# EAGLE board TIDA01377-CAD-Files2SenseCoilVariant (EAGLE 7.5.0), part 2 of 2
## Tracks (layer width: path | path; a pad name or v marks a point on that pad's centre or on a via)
ADJ
  Top 0.254: R10.2 107.83,35.93 R9.1 | 107.9,35.92 R9.1 | U1.4 107.82,35.17 107.82,35.92 R9.1
AUXVCC1  (via drill 0.2, 0.4)
  Top 0.254: MSP430F67791A.124 120.01,99.28 v121.26,98.03 | v128.51,96.62 C26.1 | C27.1 130.66,94.22 v131.51,93.38
  Top 0.406: C26.1 128.51,93.88 128.86,94.22 C27.1
  Top 0.813: 139.8,90.03 SV1.6
  Bottom 0.254: v128.51,96.62 122.66,96.62 v121.26,98.03
  Bottom 0.61: v131.51,93.38 131.47,93.34 137.36,93.34 SV1.6
AUXVCC2  (via drill 0.2, 0.6)
  Top 0.254: v120.26,98.12 119.51,98.88 MSP430F67791A.123 119.51,108.75 118.59,109.67 114.91,109.67 v114.53,110.05 | C24.1 v125.51,95.62 | v90.02,126.84 88.86,126.84 C58.1 87.27,126.8 R4.2
  Top 0.406: C24.1 125.51,94.38 125.66,94.22 C25.1
  Bottom 0.254: v125.51,95.62 122.76,95.62 v120.26,98.12 | v90.02,126.84 90.04,126.86 107.08,126.86 108.61,125.34 108.61,121.99 109.42,121.17 109.42,118.46 114.53,113.35 v114.53,110.05
  Bottom 0.61: v125.51,95.62 137.61,95.62 SV1.4
AUXVCC3  (via drill 0.3, 0.4)
  Top 0.254: C43.1 128.13,106 | MSP430F67791A.3 124.76,103.38 127.41,106.03 C43.1 | C43.1 128.01,105.88 128.16,106.03 C44.1 130.16,106.03 v131.51,107.38 | v142.76,102.12 142.76,98.62 145.31,96.07 SV1.2 148.51,90.47 D44.C
  Bottom 0.254: v131.51,107.38 138.81,107.38 142.71,103.47 142.71,102.17 v142.76,102.12 142.81,102.07
AVCC
  Top 0.254: 117.76,94.62 117.86,94.53 C29.1 | 118.01,95.88 117.96,95.83 C31.1 | MSP430F67791A.121 118.51,99.2 118.01,98.7 118.01,95.83 C31.1 | C31.1 117.81,95.83 117.76,95.88 117.91,96.03
  Top 0.406: C29.1 118.01,94.62 117.91,94.72
  Top 0.61: 117.91,94.72 C31.1 | 117.86,94.53 117.86,89.22 119.2,87.89 R36.2
BTN1  (via drill 0.6)
  Top 0.254: MSP430F67791A.7 124.86,105.38 125.19,105.71 125.19,111.34 127.23,113.38 v128.83,113.38 | v136.51,115.88 136.51,125.22 139.56,128.28 R53.2
  Top 0.406: R53.2 139.56,137.29 DBTN1.2
  Bottom 0.254: v128.83,113.38 134.01,113.38 v136.51,115.88 | 140.01,137.74 DBTN1.2
BTN2
  Top 0.254: MSP430F67791A.6 125.1,104.88 125.96,105.73 125.96,110.63 127.33,112 130.22,112 133.6,115.38 133.6,115.41 135.28,117.08 135.28,130.98 133.83,132.43 131.94,132.43 R50.2 131.89,136.36 DBTN2.2
COILS  (via drill 0.36 pad 0.58, 1.02 pad 1.52)
  Top 0.254: R12.2 v118.44,29.86 118.49,29.91 139.16,29.91 151.41,42.16 151.41,139.21 144.57,146.04 144.57,153.64 144.5,153.64 141.24,153.66 138.11,154.52 135.31,156.16 133.04,158.47 131.44,161.28 130.62,164.4 130.65,167.62 131.5,170.72 133.12,173.49 135.4,175.74 138.18,177.32 141.27,178.13 144.46,178.11 147.53,177.26 150.27,175.66 152.5,173.4 154.06,170.65 154.86,167.59 154.84,164.44 154,161.4 152.41,158.69 150.18,156.48 147.46,154.94 144.43,154.15 141.31,154.17 138.31,155 135.62,156.57 133.44,158.78 131.91,161.47 131.13,164.47 131.15,167.55 131.97,170.52 133.53,173.18 135.71,175.34 138.38,176.85 141.34,177.62 144.39,177.6 147.33,176.79 149.96,175.25 152.09,173.09 153.59,170.45 154.35,167.52 154.33,164.5 153.53,161.59 152.01,159 149.87,156.89 147.26,155.41 144.36,154.66 141.38,154.68 138.5,155.47 135.94,156.97 133.85,159.09 132.39,161.67 131.64,164.53 131.66,167.49 132.44,170.33 133.93,172.87 136.03,174.93 138.58,176.38 141.41,177.11 144.33,177.09 147.14,176.32 149.65,174.84 151.69,172.78 153.12,170.25 153.84,167.46 153.82,164.57 153.06,161.79 151.6,159.31 149.56,157.3 147.06,155.88 144.3,155.16 141.44,155.18 138.7,155.94 136.25,157.38 134.26,159.4 132.86,161.86 132.15,164.6 132.17,167.42 132.92,170.13 134.34,172.55 136.34,174.52 138.77,175.9 141.47,176.6 144.26,176.58 146.94,175.84 149.33,174.44 151.28,172.46 152.64,170.06 153.34,167.39 153.31,164.63 152.58,161.99 151.19,159.62 149.24,157.7 146.87,156.36 144.23,155.67 141.51,155.69 138.89,156.41 136.56,157.79 134.66,159.71 133.33,162.06 132.66,164.67 132.68,167.35 133.39,169.94 134.75,172.24 136.65,174.12 138.97,175.43 141.54,176.1 144.19,176.07 146.75,175.37 149.02,174.03 150.87,172.15 152.17,169.86 152.83,167.32 152.81,164.7 152.11,162.18 150.79,159.94 148.93,158.11 146.67,156.83 144.16,156.18 141.58,156.2 139.09,156.89 136.87,158.19 135.07,160.03 133.81,162.26 133.16,164.73 133.19,167.29 133.87,169.74 135.15,171.93 136.96,173.71 139.16,174.96 141.61,175.59 144.13,175.57 146.55,174.9 148.71,173.62 150.47,171.84 151.7,169.67 152.32,167.25 152.3,166.01 v151.74,166.01
  Top 0.254: 115.17,32.38 R13.2 115.15,32.4 v118.44,32.4 130.38,32.4 131.24,33.27 131.24,36.17 131.95,36.88 134.6,36.9 137.73,37.76 140.53,39.4 142.8,41.7 144.4,44.51 145.22,47.64 145.19,50.86 144.34,53.96 142.72,56.73 140.44,58.98 137.66,60.56 134.57,61.37 131.38,61.34 128.31,60.5 125.57,58.89 123.34,56.63 121.78,53.88 120.98,50.83 121,47.67 121.84,44.64 123.43,41.92 125.66,39.72 128.38,38.17 131.41,37.38 134.53,37.4 137.53,38.23 140.22,39.8 142.4,42.01 143.93,44.71 144.71,47.7 144.69,50.79 143.87,53.76 142.31,56.41 140.13,58.57 137.46,60.09 134.5,60.86 131.44,60.84 128.51,60.03 125.88,58.49 123.75,56.32 122.25,53.69 121.49,50.76 121.51,47.74 122.31,44.83 123.83,42.23 125.97,40.13 128.58,38.64 131.48,37.89 134.46,37.91 137.34,38.7 139.9,40.21 141.99,42.33 143.45,44.9 144.2,47.77 144.18,50.72 143.39,53.56 141.91,56.1 139.81,58.16 137.26,59.61 134.43,60.35 131.51,60.33 128.7,59.55 126.19,58.08 124.15,56.01 122.72,53.49 122,50.69 122.02,47.8 122.78,45.03 124.24,42.55 126.28,40.53 128.78,39.12 131.54,38.4 134.4,38.42 137.14,39.18 139.59,40.62 141.58,42.64 142.98,45.1 143.69,47.84 143.67,50.66 142.92,53.37 141.5,55.79 139.5,57.76 137.07,59.14 134.37,59.84 131.58,59.82 128.9,59.08 126.5,57.67 124.56,55.7 123.2,53.3 122.5,50.62 122.52,47.87 123.26,45.22 124.65,42.86 126.6,40.94 128.97,39.59 131.61,38.91 134.33,38.93 136.95,39.65 139.28,41.02 141.18,42.95 142.51,45.3 143.18,47.9 143.16,50.59 142.45,53.17 141.09,55.48 139.19,57.35 136.87,58.66 134.3,59.33 131.65,59.31 129.09,58.61 126.82,57.27 124.97,55.39 123.67,53.1 123.01,50.56 123.03,47.94 123.73,45.42 125.05,43.17 126.91,41.34 129.17,40.06 131.68,39.41 134.26,39.44 136.75,40.12 138.97,41.43 140.77,43.26 142.03,45.49 142.68,47.97 142.65,50.52 141.97,52.98 140.69,55.17 138.88,56.95 136.68,58.19 134.23,58.83 131.71,58.8 129.29,58.13 127.13,56.86 125.37,55.08 124.14,52.9 123.52,50.49 123.54,48 124.2,45.61 125.46,43.48 127.22,41.75 129.36,40.54 131.74,39.92 134.2,39.94 136.55,40.6 138.66,41.84 140.36,43.57 141.56,45.69 142.17,48.04 142.15,50.45 141.5,52.78 140.28,54.85 138.57,56.54 136.48,57.72 134.16,58.32 131.78,58.3 129.49,57.66 127.44,56.45 125.78,54.76 124.62,52.71 124.03,50.42 124.05,48.07 124.68,45.81 125.87,43.8 127.53,42.16 129.56,41.01 131.81,40.43 134.13,40.45 136.36,41.07 138.34,42.24 139.96,43.89 141.09,45.89 141.66,48.1 141.64,50.39 141.03,52.58 139.87,54.54 138.25,56.13 136.28,57.24 134.1,57.81 131.85,57.79 129.68,57.19 127.75,56.05 126.19,54.45 125.09,52.51 124.54,50.36 124.56,48.14 125.15,46.01 126.27,44.11 127.84,42.56 129.76,41.48 131.88,40.94 134.06,40.96 136.16,41.54 138.03,42.65 139.55,44.2 140.61,46.08 141.15,48.17 141.13,50.32 140.55,52.39 139.47,54.23 137.94,55.73 136.09,56.77 134.03,57.3 131.91,57.28 129.88,56.71 128.06,55.64 126.59,54.14 125.56,52.31 125.04,50.29 125.06,48.21 125.62,46.2 126.68,44.42 128.16,42.97 129.95,41.96 131.94,41.45 133.99,41.47 135.96,42.02 137.72,43.06 139.14,44.51 140.14,46.28 140.64,48.24 140.62,50.25 140.08,52.19 139.06,53.92 137.63,55.32 135.89,56.3 133.96,56.79 131.98,56.77 130.07,56.24 128.38,55.23 127,53.83 126.04,52.12 125.55,50.22 125.57,49.25 v126.13,49.25 v126.13,49.24
  Top 0.254: R11.2 118.36,27.25 v118.44,27.32 | v124.1,13.15 v124.1,13.14 123.54,13.14 123.52,11.9 124.14,9.49 125.37,7.31 127.13,5.53 129.29,4.26 131.71,3.59 134.23,3.57 136.68,4.2 138.88,5.45 140.69,7.22 141.97,9.41 142.65,11.87 142.68,14.42 142.03,16.9 140.77,19.13 138.97,20.96 136.75,22.27 134.26,22.95 131.68,22.98 129.17,22.32 126.91,21.05 125.05,19.22 123.73,16.97 123.03,14.45 123.01,11.83 123.67,9.29 124.97,7 126.82,5.12 129.09,3.79 131.65,3.08 134.3,3.06 136.87,3.73 139.19,5.04 141.09,6.91 142.45,9.22 143.16,11.8 143.18,14.49 142.51,17.09 141.18,19.44 139.28,21.37 136.95,22.74 134.33,23.46 131.61,23.48 128.97,22.8 126.6,21.45 124.65,19.53 123.26,17.17 122.52,14.52 122.5,11.77 123.2,9.1 124.56,6.69 126.5,4.72 128.9,3.31 131.58,2.57 134.37,2.55 137.07,3.25 139.5,4.63 141.5,6.6 142.92,9.02 143.67,11.73 143.69,14.55 142.98,17.29 141.58,19.75 139.59,21.77 137.14,23.21 134.4,23.97 131.54,23.99 128.78,23.27 126.28,21.86 124.24,19.84 122.78,17.36 122.02,14.59 122,11.7 122.72,8.9 124.15,6.38 126.19,4.31 128.7,2.84 131.51,2.06 134.43,2.04 137.26,2.78 139.81,4.23 141.91,6.29 143.39,8.83 144.18,11.67 144.2,14.62 143.45,17.49 141.99,20.06 139.9,22.18 137.34,23.69 134.46,24.48 131.48,24.5 128.58,23.75 125.97,22.27 123.83,20.16 122.31,17.56 121.51,14.65 121.49,11.63 122.25,8.7 123.75,6.07 125.88,3.9 128.51,2.36 131.44,1.55 134.5,1.53 137.46,2.3 140.13,3.82 142.31,5.98 143.87,8.63 144.69,11.6 144.71,14.69 143.93,17.68 142.4,20.38 140.22,22.59 137.53,24.16 134.53,24.99 131.41,25.01 128.38,24.22 125.66,22.67 123.43,20.47 121.84,17.76 121,14.72 120.98,11.57 121.78,8.51 123.34,5.76 125.57,3.5 128.31,1.89 131.38,1.05 134.57,1.03 137.66,1.83 140.44,3.41 142.72,5.66 144.34,8.43 145.19,11.54 145.22,14.76 144.4,17.88 142.8,20.69 140.53,22.99 137.73,24.63 134.6,25.5 131.34,25.52 131.27,25.52 131.27,26.53 131.72,26.99 v132.48,26.99
  Bottom 0.254: v120.47,27.32 120.47,13.14 120.49,11.5 121.36,8.34 123.02,5.51 125.35,3.21 128.19,1.59 131.34,0.77 134.6,0.79 137.73,1.65 140.53,3.29 142.8,5.6 144.4,8.41 145.22,11.53 145.19,14.75 144.34,17.85 142.72,20.62 140.44,22.87 137.66,24.46 134.57,25.26 131.38,25.24 128.31,24.4 125.57,22.79 123.34,20.53 121.78,17.78 120.98,14.72 121,11.57 121.84,8.53 123.43,5.82 125.66,3.62 128.38,2.07 131.41,1.28 134.53,1.3 137.53,2.13 140.22,3.7 142.4,5.91 143.93,8.61 144.71,11.6 144.69,14.69 143.87,17.66 142.31,20.31 140.13,22.47 137.46,23.98 134.5,24.75 131.44,24.73 128.51,23.92 125.88,22.38 123.75,20.22 122.25,17.58 121.49,14.66 121.51,11.63 122.31,8.73 123.83,6.13 125.97,4.02 128.58,2.54 131.48,1.79 134.46,1.81 137.34,2.6 139.9,4.11 141.99,6.22 143.45,8.8 144.2,11.66 144.18,14.62 143.39,17.46 141.91,20 139.81,22.06 137.26,23.51 134.43,24.25 131.51,24.22 128.7,23.45 126.19,21.98 124.15,19.91 122.72,17.39 122,14.59 122.02,11.7 122.78,8.92 124.24,6.44 126.28,4.43 128.78,3.02 131.54,2.3 134.4,2.32 137.14,3.07 139.59,4.51 141.58,6.54 142.98,9 143.69,11.73 143.67,14.55 142.92,17.27 141.5,19.69 139.5,21.66 137.07,23.04 134.37,23.74 131.58,23.72 128.9,22.98 126.5,21.57 124.56,19.6 123.2,17.19 122.5,14.52 122.52,11.77 123.26,9.12 124.65,6.76 126.6,4.84 128.97,3.49 131.61,2.8 134.33,2.82 136.95,3.55 139.28,4.92 141.18,6.85 142.51,9.19 143.18,11.8 143.16,14.49 142.45,17.07 141.09,19.38 139.19,21.25 136.87,22.56 134.3,23.23 131.65,23.21 129.09,22.5 126.82,21.16 124.97,19.29 123.67,17 123.01,14.46 123.03,11.84 123.73,9.32 125.05,7.07 126.91,5.24 129.17,3.96 131.68,3.31 134.26,3.33 136.75,4.02 138.97,5.33 140.77,7.16 142.03,9.39 142.68,11.87 142.65,14.42 141.97,16.87 140.69,19.06 138.88,20.84 136.68,22.09 134.23,22.72 131.71,22.7 129.29,22.03 127.13,20.76 125.37,18.97 124.14,16.8 123.52,14.39 123.54,13.14 v124.1,13.14 v124.1,13.15
  Bottom 0.254: v120.47,27.32 v118.44,27.32 | v120.47,27.32 | v151.74,166.01 152.3,166.01 152.32,164.77 151.7,162.35 150.47,160.18 148.71,158.4 146.55,157.12 144.13,156.45 141.61,156.43 139.16,157.07 136.96,158.31 135.15,160.09 133.87,162.28 133.19,164.74 133.16,167.29 133.81,169.76 135.07,172 136.87,173.83 139.09,175.13 141.58,175.82 144.16,175.84 146.67,175.19 148.93,173.91 150.79,172.09 152.11,169.84 152.81,167.32 152.83,164.7 152.17,162.16 150.87,159.87 149.02,157.99 146.75,156.65 144.19,155.95 141.54,155.93 138.97,156.59 136.65,157.91 134.75,159.78 133.39,162.09 132.68,164.67 132.66,167.35 133.33,169.96 134.66,172.31 136.56,174.23 138.89,175.61 141.51,176.33 144.23,176.35 146.87,175.67 149.24,174.32 151.19,172.4 152.58,170.03 153.31,167.39 153.34,164.63 152.64,161.96 151.28,159.56 149.33,157.58 146.94,156.18 144.26,155.44 141.47,155.42 138.77,156.12 136.34,157.5 134.34,159.47 132.92,161.89 132.17,164.6 132.15,167.42 132.86,170.16 134.26,172.62 136.25,174.64 138.7,176.08 141.44,176.84 144.3,176.86 147.06,176.14 149.56,174.72 151.6,172.71 153.06,170.23 153.82,167.45 153.84,164.57 153.12,161.77 151.69,159.25 149.65,157.18 147.14,155.71 144.33,154.93 141.41,154.91 138.58,155.65 136.03,157.09 133.93,159.16 132.44,161.69 131.66,164.53 131.64,167.49 132.39,170.35 133.85,172.93 135.94,175.05 138.5,176.55 141.38,177.34 144.36,177.37 147.26,176.61 149.87,175.13 152.01,173.02 153.53,170.43 154.33,167.52 154.35,164.5 153.59,161.57 152.09,158.93 149.96,156.77 147.33,155.23 144.39,154.42 141.34,154.4 138.38,155.17 135.71,156.69 133.53,158.84 131.97,161.5 131.15,164.47 131.13,167.56 131.91,170.55 133.44,173.24 135.62,175.45 138.31,177.03 141.31,177.85 144.43,177.88 147.46,177.09 150.18,175.54 152.41,173.33 154,170.62 154.84,167.59 154.86,164.43 154.06,161.37 152.5,158.62 150.27,156.37 147.53,154.76 144.46,153.91 141.27,153.89 138.18,154.7 135.4,156.28 133.12,158.53 131.5,161.3 130.65,164.4 130.62,167.62 131.44,170.75 133.04,173.56 135.31,175.86 138.11,177.5 141.24,178.36 144.5,178.38 147.65,177.56 150.49,175.94 152.82,173.65 154.48,170.82 155.35,167.65 155.37,166.01 155.37,151.83 155.37,40.1 142.26,26.99 v132.48,26.99
  Bottom 0.254: v126.13,49.24 v126.13,49.25 125.57,49.25 125.55,48.27 126.04,46.38 127,44.67 128.38,43.26 130.07,42.25 131.98,41.72 133.96,41.7 135.89,42.2 137.63,43.17 139.06,44.58 140.08,46.3 140.62,48.24 140.64,50.26 140.14,52.22 139.14,53.98 137.72,55.44 135.96,56.48 133.99,57.03 131.94,57.05 129.95,56.53 128.16,55.52 126.68,54.08 125.62,52.29 125.06,50.29 125.04,48.2 125.56,46.18 126.59,44.35 128.06,42.85 129.88,41.78 131.91,41.21 134.03,41.19 136.09,41.72 137.94,42.77 139.47,44.26 140.55,46.11 141.13,48.17 141.15,50.32 140.61,52.41 139.55,54.3 138.03,55.84 136.16,56.95 134.06,57.53 131.88,57.55 129.76,57.01 127.84,55.93 126.27,54.39 125.15,52.49 124.56,50.35 124.54,48.14 125.09,45.98 126.19,44.04 127.75,42.45 129.68,41.31 131.85,40.71 134.1,40.69 136.28,41.25 138.25,42.36 139.87,43.95 141.03,45.91 141.64,48.11 141.66,50.39 141.09,52.61 139.96,54.61 138.34,56.25 136.36,57.42 134.13,58.04 131.81,58.06 129.56,57.48 127.53,56.34 125.87,54.7 124.68,52.68 124.05,50.42 124.03,48.07 124.62,45.79 125.78,43.73 127.44,42.04 129.49,40.83 131.78,40.2 134.16,40.18 136.48,40.77 138.57,41.95 140.28,43.64 141.5,45.71 142.15,48.04 142.17,50.46 141.56,52.8 140.36,54.92 138.66,56.66 136.55,57.9 134.2,58.55 131.74,58.57 129.36,57.95 127.22,56.74 125.46,55.01 124.2,52.88 123.54,50.49 123.52,48 124.14,45.59 125.37,43.42 127.13,41.63 129.29,40.36 131.71,39.69 134.23,39.67 136.68,40.3 138.88,41.55 140.69,43.33 141.97,45.52 142.65,47.97 142.68,50.52 142.03,53 140.77,55.23 138.97,57.06 136.75,58.37 134.26,59.06 131.68,59.08 129.17,58.43 126.91,57.15 125.05,55.32 123.73,53.08 123.03,50.55 123.01,47.94 123.67,45.39 124.97,43.11 126.82,41.23 129.09,39.89 131.65,39.18 134.3,39.16 136.87,39.83 139.19,41.14 141.09,43.02 142.45,45.32 143.16,47.91 143.18,50.59 142.51,53.2 141.18,55.54 139.28,57.47 136.95,58.84 134.33,59.57 131.61,59.59 128.97,58.9 126.6,57.55 124.65,55.63 123.26,53.27 122.52,50.62 122.5,47.87 123.2,45.2 124.56,42.79 126.5,40.82 128.9,39.41 131.58,38.67 134.37,38.65 137.07,39.36 139.5,40.74 141.5,42.7 142.92,45.12 143.67,47.84 143.69,50.66 142.98,53.39 141.58,55.86 139.59,57.88 137.14,59.32 134.4,60.07 131.54,60.09 128.78,59.38 126.28,57.96 124.24,55.95 122.78,53.47 122.02,50.69 122,47.8 122.72,45 124.15,42.48 126.19,40.41 128.7,38.94 131.51,38.17 134.43,38.14 137.26,38.88 139.81,40.33 141.91,42.39 143.39,44.93 144.18,47.77 144.2,50.73 143.45,53.59 141.99,56.17 139.9,58.28 137.34,59.79 134.46,60.58 131.48,60.6 128.58,59.85 125.97,58.37 123.83,56.26 122.31,53.66 121.51,50.76 121.49,47.73 122.25,44.81 123.75,42.17 125.88,40.01 128.51,38.47 131.44,37.66 134.5,37.64 137.46,38.41 140.13,39.92 142.31,42.08 143.87,44.73 144.69,47.7 144.71,50.79 143.93,53.78 142.4,56.48 140.22,58.69 137.53,60.26 134.53,61.09 131.41,61.11 128.38,60.32 125.66,58.77 123.43,56.57 121.84,53.86 121,50.82 120.98,47.67 121.78,44.61 123.34,41.86 125.57,39.6 128.31,37.99 131.38,37.15 134.57,37.13 137.66,37.94 140.44,39.52 142.72,41.77 144.34,44.54 145.19,47.64 145.22,50.86 144.4,53.98 142.8,56.79 140.53,59.1 137.73,60.74 134.6,61.6 131.34,61.62 128.19,60.8 125.35,59.18 123.02,56.88 121.36,54.05 120.49,50.89 120.47,50.87 120.47,49.25 v120.47,27.32
COM0  (via drill 0.2)
  Top 0.254: MSP430F67791A.22 121.01,112.88 v113.51,120.38 | LCD1.COM0 94.38,171.5 v109.26,156.62
  Bottom 0.254: v113.51,120.38 113.51,152.38 v109.26,156.62
COM1  (via drill 0.2)
  Top 0.254: MSP430F67791A.23 121.51,113.38 v114.51,120.38 | v109.26,158.12 109.26,158.15 96.62,170.78 96.62,171.46 LCD1.COM1
  Bottom 0.254: v114.51,120.38 114.51,152.88 v109.26,158.12
COM2  (via drill 0.2)
  Top 0.254: MSP430F67791A.24 122.01,113.88 v115.51,120.38 | LCD1.COM2 99.2,169.68 v109.26,159.62
  Bottom 0.254: v115.51,120.38 115.51,153.38 v109.26,159.62
COM3  (via drill 0.2)
  Top 0.254: MSP430F67791A.25 122.51,114.38 v116.51,120.38 | v109.26,161.12 109.26,161.19 101.7,168.75 101.7,171.46 LCD1.COM3
  Bottom 0.254: v116.51,120.38 116.51,153.88 v109.26,161.12
DRESET  (via drill 0.36)
  Top 0.254: v49.01,129.88 49.51,129.38 89.51,129.38 91.01,127.88 91.01,111.77 v91.03,111.75 | MSP430F67791A.102 106.51,102.38 v104.63,100.5
  Bottom 0.254: JP5.2 27.99,136.81 42.08,136.81 v49.01,129.88 | v104.63,100.5 96.38,100.5 91.13,105.75 91.13,111.65 v91.03,111.75
DRV4GND
  Top 0.254: MSP430F67791A.95 95.09,105.88 90.63,101.41 90.63,84.78 90.09,84.24 67.21,84.24 66.57,84.88 66.57,85.97 65.7,86.84 U4GND.1
DRV5GND
  Top 0.254: MSP430F67791A.93 94.16,106.88 89.46,102.18 89.46,88.28 87.98,86.81 U5GND.1
DRV6GND
  Top 0.254: MSP430F67791A.88 93.51,109.38 87.35,103.22 87.35,95.98 85.77,94.4 78.36,94.4 75.39,97.38 75.39,100.53 73.33,102.58 68.2,102.58 67.41,101.8 67.41,100.67 U6GND.1
DRV456OUTA  (via drill 0.5, 0.6)
  Top 0.254: MSP430F67791A.89 93.74,108.88 87.93,103.06 87.93,94.66 86.76,93.49 78.36,93.49 v78.1,93.23 78.03,93.31 75.84,93.31 75.79,93.36 75.77,93.36 73.73,95.39 73.73,99.05 73.19,99.6 U6OUT.1 | U5OUT.1 83.44,90.44 v84.4,89.48
  Top 0.305: U4OUT.1 59.67,83.44 v59.97,83.15 | 79.82,90.42 U5OUT.1
  Bottom 0.254: v59.97,83.15 75.16,83.15 | v84.4,89.48 84.4,84.09 83.46,83.15 75.16,83.15 | 75.16,83.15 75.61,83.61 75.61,92.35 76.58,93.31 78.03,93.31 v78.1,93.23
DRV456OUTB
  Top 0.254: MSP430F67791A.94 94.62,106.38 89.99,101.74 89.99,85.13 89.56,84.7 69.59,84.7 69.19,85.11 U$8.3
DRVOUT4  (via drill 0.5, 0.6)
  Top 0.254: U$8.1 | 70.86,83.79 65.56,83.79 65.02,84.32 65.02,85.21 | 70.86,83.79 109.75,83.79 v110.08,84.12 | v114.45,106.29 118.31,106.29 v118.36,106.24 | v121.54,106.24 122.2,106.24 122.33,106.38 MSP430F67791A.9 | 68.03,79.15 R17.1 69.75,79.15 C12.1 69.67,79.23 69.67,80.87 70.15,81.35 70.15,83.08 70.86,83.79
  Top 0.305: U$8.1 68.17,85.36 v68.02,85.21 | v65.48,85.21 65.02,85.21
  Bottom 0.254: v110.08,84.12 110.08,101.92 v114.45,106.29 | v118.36,106.24 v121.54,106.24
  Bottom 0.305: v68.02,85.21 v65.48,85.21
DRVOUT5  (via drill 0.6)
  Top 0.254: 86.15,91.58 v86.21,91.53 86,91.74 72.06,91.74 71.17,90.85 71.17,89.3 71.65,88.81 72.61,88.81 C14.1 72.58,88.64 72.58,86.99 R16.1 71.55,86.94 | MSP430F67791A.10 123.78,106.85 122.12,106.85 v121.51,107.46 | v118.26,107.46 115.57,107.46 115.34,107.69 114.5,107.69 v114.48,107.66
  Top 0.305: U$8.2 68.68,86.66 68.96,86.94 71.55,86.94
  Bottom 0.254: v86.21,91.53 90.32,91.53 97,84.85 108.71,84.85 109.55,85.69 109.55,102.73 v114.48,107.66 | v121.51,107.46 v118.26,107.46
DRVOUT6  (via drill 0.6)
  Top 0.254: v117.96,108.63 113.61,108.63 v113.59,108.6 | U$8.5 69.68,92.96 R15.1 69.63,93.03 71.63,93.03 72.31,92.35 87.96,92.35 v88.19,92.57 | MSP430F67791A.11 123.02,107.38 v121.79,108.6
  Top 0.305: R15.1 67.82,93.02 C15.1
  Bottom 0.254: v117.96,108.63 117.98,108.6 v121.79,108.6 | v113.59,108.6 113.59,108.55 108.61,103.57 108.61,93.56 107.11,92.07 105.26,92.07 104.75,92.57 v88.19,92.57
DRVPOWER1
  Top 0.61: R1.1 28.88,191.68 28.88,190.44 28.37,189.93 DRV_U$7.1 22.85,189.9 U$7.1 18.82,189.9 18.57,190.16 18.57,193.96 C1.1
DRVPOWER4  (via drill 0.5)
  Top 0.254: v60.93,92.45 64.11,92.45 66.25,90.3 R68.2
  Top 0.61: 59.25,89.58 R45.1 | R45.1 59.11,89.8 | v60.93,92.45 60.45,91.96 C52.1 59.5,91.14 59.1,90.75 59.1,89.44 R45.1 | U$4.1 59.24,89.3 R45.1
  Bottom 0.305: 71.34,100.16 R64.1
  Bottom 0.61: 82.14,95.72 85.14,95.72 87.32,97.91 DRV-I1.1 | C54.1 81.03,88.37 U$5.1 80.62,89.94 80.67,89.98 R47.1 80.31,90.56 80.31,93.89 82.14,95.72 | 71.34,100.16 U$6.1 68.74,100.72 C55.1 62.83,100.72 60.96,98.85 60.96,92.47 v60.93,92.45 | R64.1 71.55,100.17 73.05,100.17 74.88,98.33 74.88,96.16 75.32,95.72 82.14,95.72
DRVU7  (via drill 0.6)
  Top 0.254: R1.2 27.04,192.87 28.55,194.38 32.05,194.38 39.14,187.29 39.14,163.09 v57.4,144.82 | MSP430F67791A.20 121.69,111.88 v121.66,111.85
  Top 0.61: U$7.2 26.97,191.8 R1.2
  Bottom 0.254: v57.4,144.82 105.05,144.82 109.47,140.4 109.47,123.31 120.93,111.85 v121.66,111.85
DTCK  (via drill 0.36)
  Top 0.254: v50.01,130.38 50.51,129.88 89.76,129.88 91.51,128.12 91.51,112.88 v91.88,112.5 | MSP430F67791A.101 105.51,102.88 v103.88,101.25
  Bottom 0.254: JP6.2 27.99,139.35 34.88,139.35 36.67,137.56 42.83,137.56 v50.01,130.38 | v103.88,101.25 96.68,101.25 91.72,106.21 91.72,112.33 v91.88,112.5
DTDI  (via drill 0.36)
  Top 0.254: v52.01,131.38 52.51,130.88 90.26,130.88 92.51,128.62 92.51,114.7 v93.31,113.9 | MSP430F67791A.99 103.51,103.88 v102.38,102.75
  Bottom 0.254: JP8.2 28.08,144.34 32.84,144.34 35.13,142.05 41.33,142.05 v52.01,131.38 | v102.38,102.75 102.34,102.71 98.02,102.71 93.38,107.34 93.38,113.82 v93.31,113.9
DTDO  (via drill 0.36)
  Top 0.254: v53.01,131.88 53.51,131.38 90.51,131.38 93.01,128.88 93.01,115.57 v93.93,114.65 | MSP430F67791A.98 102.51,104.38 v101.63,103.5
  Bottom 0.254: JP9.2 27.99,146.97 31.74,146.97 35.64,143.07 39.67,143.07 | 39.67,143.07 39.7,143.07 | 39.67,143.07 39.69,143.06 41.83,143.06 v53.01,131.88 | v101.63,103.5 101.55,103.42 98.5,103.42 94.13,107.79 94.13,114.44 v93.93,114.65
DTMS  (via drill 0.36)
  Top 0.254: v51.01,130.88 51.51,130.38 90.01,130.38 92.01,128.38 92.01,113.88 v92.63,113.25 | MSP430F67791A.100 104.51,103.38 v103.13,102
  Bottom 0.254: JP7.2 27.99,141.89 33.84,141.89 37.17,138.56 43.33,138.56 v51.01,130.88 | v92.63,113.25 92.63,106.49 97.23,101.9 103.03,101.9 v103.13,102
DVCC  (via drill 0.36, 0.36 pad 0.58, 0.5, 0.6)
  Top 0.254: MSP430F67791A.126 121.01,99.78 121.91,98.88 C35.1 | R50.1 130.19,134.54 129.03,135.7 129.03,137.99 130.22,139.18 135.96,139.18 | 135.96,139.18 139.7,139.18 141.98,136.9 | R53.1 137.86,137.29 135.96,139.18
  Top 0.305: R51.1 33.67,147.06 26.09,154.59 JP10.2
  Top 0.406: 123.51,97.38 C33.1 124.01,97.28
  Top 0.61: 124.01,97.28 v124.01,87.88 121.88,87.88 | C33.1 C35.1 | 58.4,173.38 v58.5,173.28 R54.1 | R55.1 v63.95,173.28 | R56.1 v69.03,173.28 | R57.1 v74.11,173.28 | R58.1 v86.81,173.28 | R59.1 v91.89,173.28 | R60.1 v96.97,173.28 | R61.1 v102.31,173.28 | v81.89,116.55 81.89,116.62 81.09,117.42
  Top 0.813: DVCC.1 DVCC.2 DVCC.3 DVCC.4 | 121.88,87.88 R36.1 | 124.05,87.92 v124.01,87.88 131.11,87.88 136.93,93.69 136.93,97.8 142.01,102.88 142.01,106.09 v141.98,106.11 | 81.09,117.42 v81.09,127.43 | v81.09,127.43 | v103.33,188.79 114.24,177.88 v114.24,161.03 | v141.98,118.18 141.98,136.9 141.96,136.92 141.96,138.9 140.98,139.88 140.82,140.05 140.79,140.07 v124.56,140.07
  Bottom 0.61: v102.31,173.28 v96.97,173.28 v91.89,173.28 v86.81,173.28 v74.11,173.28 v69.03,173.28 v63.95,173.28 v58.5,173.28 | R66.2 87.27,114.95 86.54,115.69 82.75,115.69 v81.89,116.55
  Bottom 0.813: 47.01,154.05 47.01,171.69 48.61,173.3 48.63,173.28 50.43,173.28 | v81.09,127.43 81.09,128.97 77.69,132.38 56.51,132.38 47.01,141.88 47.01,154.05 | JP10.2 24.18,154.57 24.17,154.56 | v141.98,106.11 v141.98,118.18 | 24.33,154.73 46.05,154.73 46.19,154.87 | v103.33,188.79 62.94,188.79 | 62.94,188.79 55.47,188.79 51.61,184.93 51.61,174.28 | v58.5,173.28 50.43,173.28 | 46.19,154.87 46.91,155.59 | 46.96,153.87 46.18,154.65 46.33,154.65 46.37,154.69 | 47.01,154.05 46.37,154.69 | 46.37,154.69 46.19,154.87 | DVCC.1 63.13,188.98 62.94,188.79 | 51.18,173.85 52.02,173.85 | 51.61,174.54 51.61,174.46 50.71,173.56 | 50.43,173.28 50.42,173.27 | 51.59,174.57 51.74,174.41 | 51.74,174.41 52.78,173.37 | 50.43,173.28 50.71,173.56 | 50.71,173.56 50.89,173.56 51.18,173.85 | 51.61,174.28 51.74,174.41 | 51.61,174.28 51.18,173.85 | 51.13,173.85 51.18,173.85 | v114.24,161.03 114.24,160.45 119.73,154.96 119.73,142.18 121.84,140.07 v124.56,140.07
  Bottom 1.27: 24.33,154.73 JP10.2
DVSYS_VDSYS  (via drill 0.2, 0.4, 0.5, 0.6)
  Top 0.254: 129.26,98.9 C34.1 128.23,97.88 v126.76,97.88 | C36.1 106.28,122.75 106.81,122.75 108.05,121.5 108.41,121.5 109.27,120.64 109.27,119.62 110.01,118.89 110.01,118.88 120.51,108.44 MSP430F67791A.125 120.51,99.53 122.36,97.88 v122.51,97.88 | MSP430F67791A.69 106.51,118.88 v106.26,118.62
  Top 0.406: 129.26,98.9 130.48,98.9 v131.76,97.62 | LDC_PWR.2 47.93,128.64 v56.23,120.34
  Top 0.61: DRVPWR4.1 v89.02,120.46 | v106.26,121.62 C36.1
  Bottom 0.254: v122.51,97.88 v126.76,97.88
  Bottom 0.406: v56.23,120.34 88.9,120.34 v89.02,120.46
  Bottom 0.61: v131.76,97.62 146.23,97.62 147.04,96.82 147.04,89.65 SV1.1 | v89.02,120.46 105.67,120.46 106.26,119.88 | 106.26,119.88 v106.26,118.62 | 106.26,119.88 v106.26,121.62
EN  (via drill 0.6)
  Top 0.254: U1.6 101.91,31.59 99.36,34.13 EN_SEL.2 | AD_SEL.3 107.85,39.08 107.34,39.59 100.45,39.59 99.36,38.5 v99.36,38.34
  Top 0.406: LDIG.2 19.17,120.62 20.93,118.86 20.93,48.45 24.03,45.36 80.11,45.36 v80.13,45.38 | v99.36,38.34 EN_SEL.2
  Bottom 0.406: v80.13,45.38 92.33,45.38 v99.36,38.34
EXT
  Top 0.813: JP10.3
  Top 1.016: JTAG.4 19.39,150.78 20.67,152.06 JP10.3
GND  (via drill 0.3, 0.3 pad 0.25, 0.36, 0.4, 0.5, 0.6)
  Top 0.254: MSP430F67791A.70 108.77,118.38 108.94,118.2 108.94,115.69 v109.51,115.12 | C10.2 99.15,32.48 100.3,32.48 100.53,32.25 C11.2 100.57,31.44 101.32,31.44 101.67,31.09 U1.7 103.53,31.09 U1.9 | v122.5,118.38 MSP430F67791A.33 | MSP430F67791A.120 118.01,101.78 v118.09,101.87 | MSP430F67791A.127 121.51,102.07 v121.54,102.1 | MSP430F67791A.112 114.01,101.58 v114.27,101.85
  Top 0.406: v59.28,41.5 59.28,41.37 | 71.35,29.3 71.45,29.3 | 103.73,29.38 103.73,30.89 v103.76,30.92
  Top 0.61: C1.2 15.64,194.4 15.21,193.97 15.21,191.94 16.36,190.8 17.35,190.8 U$7.3 | 103.73,31.28 U1.9
  Top 0.813: LDIG.4 23.34,125.7 25.32,123.72 25.32,52.52 26.24,51.6 48.36,51.6 v48.38,51.58 | 59.28,41.37 59.38,41.37 71.45,29.3 71.45,29.23 72.08,28.59 101.5,28.59 102.21,29.3 C9.2
  Bottom 0.813: v59.28,41.5 49.2,51.58 v48.38,51.58
  other vias: 105.42,118.69 128.01,121.38 129.51,128.38 109.95,109.24 137.31,113.23 139.31,116.73 131.32,109.29 130.76,102.62 134.51,104.62 134.51,100.62 109.51,114.12 107.01,127.88 107.01,131.88 86.51,157.38 74.01,157.38 61.51,157.38 88.99,128.17 86.51,150.38 74.01,150.38 61.51,150.38 130.26,97.67 139.31,119.23 139.31,121.23 139.31,123.23 115.94,103.57 120.26,91.88 112.18,90.4 121.76,91.88 121.76,90.38 120.26,90.38 120.26,84.38 126.35,82.57 101.19,95.44 96.44,90.69 96.44,95.44 114.4,104.13 96.43,98.44 101.19,98.44 101.19,90.69 66.34,87.5 70.56,85.67 83.61,80.41 94.18,94.27 103.63,94.06 96.44,88.14 101.19,88.14 44.61,184.03 44.61,182.25 44.61,179.97 46.64,179.97 46.64,182.25 46.64,184.03 109.95,111.52 109.95,113.05 111.48,113.05 113.51,116.86 122.37,120.36 125.24,120.87 115.64,110.99 112.05,109.67 109.95,106.9 62.81,87.42 63.62,91.53 125.06,118.89 122.5,117.52 101.52,27.29 104.19,27.29 104.26,25.61 101.57,25.61 97.94,32.52 94.99,27.29 103.98,33.92 110.79,22.74 73.63,90.82 123.39,101.64 114.2,97.81 95.2,77.1 94.69,70.19 106.91,96.58 111.35,108.06 115.59,105.17 118.52,104.96 114.68,115.88 116.86,114.36 112.59,118.45 107.87,123.88 82.75,124.49 89.91,122.99 83.05,118.14 83.46,111.94 72.56,112.58 73.45,116.95 69.62,123.76 61.79,116.57 57.43,125.28 51.99,134.78 42.62,130.59 39.24,122.23 28.32,125.56 26.41,114.79 12.44,113.52 10.77,103.26 87.96,40.7 49.3,40.49 102.4,107.79 96.59,111.91 115.67,104.28 94.99,25.61 94.31,32.6 90.83,32.6 84.1,32.6 79.09,33.26 65.63,46.67 46.66,46.67 43.25,40.49 36.88,40.49 29.99,40.49 24.81,40.49 17.88,40.49 10.77,40.49 91.64,40.8 87.86,39.07 91.64,39.07 10.77,67.57 10.77,86.95 68.98,40.52 39.42,114.08 34.48,183.86 28.51,183.88 28.51,180.07 34.48,179.94 28.36,174.18 34.48,174.18 132.1,82.48 132.1,85.43 31.39,100.08 31.39,95.07 31.39,91.01 31.39,88.06 144.9,106.46 144.9,111.46 144.9,115.53 144.9,118.47 148.05,106.48 148.05,111.49 148.05,115.55 148.05,118.5 114.23,193.89 109.23,193.89 105.16,193.89 102.22,193.89 114.26,191.76 109.25,191.76 105.19,191.76 102.24,191.76 88.68,185.31 83.68,185.31 79.61,185.31 76.66,185.31 53.2,192.24 48.19,192.24 44.13,192.24 41.18,192.24 57.16,111.83 52.15,111.83 48.09,111.83 45.14,111.83 41.75,88.02 41.75,93.02 41.75,97.09 41.75,100.03 42.01,69.58 42.01,74.58 42.01,78.65 42.01,81.59 31.65,81.64 31.65,76.63 31.65,72.57 31.65,69.62 69.4,72.23 64.4,72.23 60.33,72.23 57.39,72.23 57.34,61.87 62.34,61.87 66.41,61.87 69.36,61.87 86.65,72.15 81.64,72.15 77.58,72.15 74.63,72.15 74.59,61.79 79.59,61.79 83.66,61.79 86.6,61.79 74.54,53.76 79.54,53.76 83.6,53.76 86.55,53.76 57.29,53.84 62.29,53.84 66.36,53.84 69.3,53.84 42.01,53.55 42.01,58.55 42.01,62.62 42.01,65.56 31.65,65.61 31.65,60.61 31.65,56.54 31.65,53.6 103.76,31.72 26.08,100.15 25.96,95.02 25.96,90.68 25.98,87.94 26.01,105.64 26.31,110.54 30.33,110.54 33.96,110.62 15.64,110.42 25.98,83.39 26.06,76.63 25.91,72.09 19.56,109.93 19.48,105.61 19.66,100.05 19.71,95.35 19.79,90.12 19.79,87.61 19.71,83.59 19.71,76.91 19.84,72.04 19.91,69.39 19.73,65.89 19.68,61.32 19.63,57.23 25.91,69.14 26.08,65.58 26.08,61.04 26.19,57.3 26.9,53.24 53.62,49.92 57.1,49.89 56.46,46.67 23.7,110.85 23.67,112.42 23.7,114.25 23.65,115.7 23.65,107.04 23.65,100.48 23.75,95.23 23.57,90.7 23.57,88.01 23.72,83.52 23.85,76.73 23.82,72.24 23.77,69.04 23.72,65.71 23.77,61.11 23.72,57.33 23.82,53.42 25.65,49.99 28.78,49.84 32.38,49.79 37.21,49.61 40.84,49.68 45.16,49.63 25.7,46.61 28.6,46.58 32.28,46.56 37.03,46.58 40.99,46.58 48.26,49.68 49.65,46.87 61.08,46.59 60.96,42.09 62.73,40.34 64.59,38.51 66.29,36.74 69.03,34.14 72.67,34.22 72.64,31.63 70.38,37.37 73.86,37.24 73.45,40.44 77.82,40.44 77.9,37.27 82.22,40.37 82.32,37.27 87.73,37.45 91.51,37.57 79.09,34.65 83.92,34.5 90.65,34.5 94.43,34.32 62.38,35.14 62.51,32.21 65.68,32.11 62.51,29.19 66.09,29.37 80.74,29.65 92.95,53.54 92.8,61.79 99.69,70.49 99.69,74.58 99.51,78.42 99.21,82 99.69,66.22 99.69,61.02 99.69,55.81 99.49,49.69 104.14,55.99 104.31,50.35 104.01,61.2 104.01,66.2 103.91,70.34 103.83,74.48 103.93,78.75 113.2,85.4 115.36,86.06 115.26,90.51 112.34,86.84 104.62,46.26 64.72,42.73 80.84,46.46 83.82,46.46 86.79,46.54 89.76,46.9 93.6,46.84 94.03,45.17 96.52,42.76 99.34,42.76 72.31,46.77 25.63,43.87 28.57,43.89 32.1,43.89 37.08,43.89 40.94,43.82 46.51,44.1 50.06,43.87 54.13,44.1 58.27,44.35 67.56,44.4 70.26,43.28 73.79,43.38 77.34,43.49 81.86,43.36 87.48,43.41 92.1,43.31
  pour Bottom: 3.66,37.79 3.66,164.89 11.88,164.89 11.88,195.7 115.11,195.7 115.11,160.65 115.11,160.6 120.5,155.21 120.5,153.43 123.42,150.51 123.42,141.14 123.72,140.83 141.7,140.83 143.76,138.78 150.37,138.78 150.37,79.19 106.4,79.19 106.4,26.31 112.44,26.31 112.44,22.14 90.88,22.14 90.88,27.58 60.88,27.58 60.88,37.79
  pour Top: 3.66,37.79 3.66,164.89 11.88,164.89 11.88,195.7 115.11,195.7 115.11,160.65 115.11,160.6 120.5,155.21 120.5,153.43 123.42,150.51 123.42,141.14 123.72,140.83 141.7,140.83 143.76,138.78 150.37,138.78 150.37,79.19 106.4,79.19 106.4,26.31 112.44,26.31 112.44,22.14 90.9,22.14 90.9,27.58 60.88,27.58 60.88,37.79
INT
  Top 1.016: JTAG.2 18.43,153.32 22.24,157.13 JP10.1
LCOM
  Top 0.254: U1.1 105.24,30.07 C9.1 106.73,29.3 108.79,27.25 110.44,27.25 LANLG.2 110.64,27.45 112.24,27.45 112.44,27.25 R11.1
LDC0851_OUT  (via drill 0.6)
  Top 0.254: MSP430F67791A.4 v121.82,103.88 | U1.5 v102.83,37.67 | v102.61,43.88 102.61,79.98 103.71,81.07 114.96,81.07 v117.6,83.71
  Top 0.406: v102.83,37.67 v102.84,37.69 | LDIG.1 18.25,117.81 18.25,46.66 21.03,43.88 21.03,43.86 22.71,42.18 57.61,42.18 59.18,43.76 66.44,43.76 68.4,41.8 100.53,41.8 v102.61,43.88
  Bottom 0.254: v117.6,83.71 117.52,83.79 117.52,98.31 117.19,98.64 117.19,103.24 117.83,103.88 v121.82,103.88
  Bottom 0.406: v102.84,37.69 102.84,43.65 v102.61,43.88 | R8.1 LDIG.1
LDC_EN_MCU  (via drill 0.6)
  Top 0.254: EN_SEL.1 101.06,37.38 v101.12,37.43 | v101.14,45.05 101.14,80.56 102.97,82.39 114.2,82.39 v114.68,82.87 | MSP430F67791A.15 122.92,109.38 121.28,111.02 119.35,111.02 v119.28,110.94
  Bottom 0.254: v119.28,110.94 117.45,110.94 116.71,110.2 116.71,84.9 v114.68,82.87 | v101.12,37.43 101.12,45.03 v101.14,45.05
LDC_VDD  (via drill 0.3 pad 0.25, 0.36 pad 0.25)
  Top 0.254: U1.8 101.86,30.59 101.42,30.14 100.57,30.14 C11.1 99.87,30.84 C10.1 99.04,30.8 | AD_SEL.1 111.25,39.9 110.06,41.09 98.19,41.09 97.66,40.56 EN_SEL.3 97.74,35.63
  Top 0.406: LED7.A 35.22,126.42 34.41,127.22 14.22,127.22 LDC_PWR.1 13.21,126 13.21,124.35 14.4,123.16 LDIG.3
  Top 0.813: LDIG.3 20.65,123.16 22.3,121.5 22.3,50.49 24.76,48.02 v56.94,48.02 | C10.1 98.99,30.75 78.48,30.75 73.53,35.7 | EN_SEL.3 73.53,35.7 | v62.71,42.77 62.71,42.49 69.49,35.7 73.53,35.7
  Bottom 0.813: v56.94,48.02 57.45,48.02 v62.71,42.77
LED1
  Top 0.254: MSP430F67791A.28 127.76,115.88 129.51,117.62 129.51,124.88 127.51,126.88 123.26,126.88 122.01,128.12 122.01,149.88 111.51,160.38 111.51,171.88 103.01,180.38 73.85,180.38 LED1.K
LED2
  Top 0.254: MSP430F67791A.27 128.01,115.38 130.01,117.38 130.01,125.12 127.76,127.38 123.51,127.38 122.51,128.38 122.51,150.12 112.01,160.62 112.01,172.12 103.26,180.88 69.27,180.88 LED2.K
LED3
  Top 0.254: MSP430F67791A.26 128.26,114.88 130.51,117.12 130.51,125.38 128.01,127.88 123.76,127.88 123.01,128.62 123.01,150.38 112.51,160.88 112.51,172.38 103.51,181.38 64.69,181.38 LED3.K
LED4
  Top 0.254: MSP430F67791A.45 119.01,145.88 110.01,154.88 110.01,171.12 102.26,178.88 90.01,178.88 88.98,177.84 LED4.K
LED5  (via drill 0.36)
  Top 0.254: MSP430F67791A.43 120.01,147.67 v118.79,148.89
  Bottom 0.254: v118.79,148.89 118.79,154.65 112.62,160.82 112.62,172.79 106.35,179.06 95.39,179.06 LED5.K
LED6  (via drill 0.36)
  Top 0.254: MSP430F67791A.44 119.51,146.47 v117.65,148.33
  Bottom 0.254: v117.65,148.33 117.65,155.03 111.86,160.82 111.86,172.33 106.32,177.87 99.28,177.87 LED6.K
LED_B
  Top 0.254: LED_B.K 85.55,179.38 102.51,179.38 110.51,171.38 110.51,159.88 120.51,149.88 MSP430F67791A.42
LEDA
  Top 0.254: MSP430F67791A.29 127.51,116.38 129.01,117.88 129.01,124.62 127.26,126.38 123.01,126.38 121.51,127.88 121.51,149.62 111.01,160.12 111.01,171.62 102.76,179.88 78.43,179.88 LED_A.K
  Bottom 0.254: 76.36,177.72 LED_A.K 76.32,177.77
LREF
  Top 0.254: U1.3 107.41,31.59 108.25,32.43 110.54,32.43 LANLG.4 113.35,32.45 R13.1
LSENSE
  Top 0.254: U1.2 107.39,31.09 108.63,29.84 110.49,29.84 LANLG.3 113.3,29.91 R12.1
N$4
  Top 0.254: R56.2 72.05,174.34 LED1.A
N$7
  Top 0.254: R55.2 66.97,174.34 LED2.A
N$10
  Top 0.254: JP4.1 27.99,136.81 22.14,136.81 21.62,137.33 R48.2
N$15  (via drill 0.6)
  Top 0.406: LED7.C 31.62,125.85 v30.53,124.76
  Bottom 0.406: v30.53,124.76 30.53,118.09 R8.2
N$16
  Top 0.254: R9.2 AD_SEL.2
N$17
  Top 0.254: R17.2 64.17,81.05 63.07,82.15 U4OUT.3
N$18
  Top 0.254: D44.A 148.54,84.02 HD1.2
N$19
  Top 0.254: R16.2 75.54,86.94 76.1,87.49 76.1,90.14 U5OUT.3
N$20
  Top 0.305: U6OUT.3 69.92,96.2 69.64,95.93 69.64,94.95 R15.2
N$21
  Top 0.254: R59.2 88.13,174.34 LED4.A
N$24
  Top 0.61: 64.21,88.62 U4GND.2 64.09,88.34 U$4.3 62.81,89.18 62.23,89.75 62.23,91.02 C52.2
N$26
  Top 0.61: U5GND.2 79.31,88.73 U$5.2
  Bottom 0.61: 79.38,88.81 U$5.2 79.13,88.56 C54.2
N$27
  Top 0.254: R60.2 93.21,174.34 LED5.A
N$28
  Top 0.61: U6GND.2 69.26,98.86 U$6.2
  Bottom 0.305: 67.59,98.89 C55.2
  Bottom 0.61: 67.59,98.89 U$6.2
N$30
  Top 0.254: R54.2 61.89,174.34 LED3.A
N$36
  Top 0.254: R61.2 98.29,174.34 LED6.A
N$41
  Top 0.61: 59.17,87.67 R45.2 59.14,87.7 59.92,87.7 60.22,87.39 U$4.2 60.48,87.38 60.48,86.71 61.37,85.81 U4OUT.2
N$43
  Top 0.61: U5OUT.2 78.09,88.79 U$5.3
  Bottom 0.61: U$5.3 78.08,90.03 R47.2
N$44
  Top 0.254: R58.2 83.05,174.34 LED_B.A
N$46
  Top 0.254: R57.2 77.13,174.34 LED_A.A
N$49
  Top 0.61: D26.A 87.06,125.21 R4.1
N$50
  Top 0.305: U$8.6 U$8.7
N$51  (via drill 0.5)
  Top 0.61: D27.A v87.22,109.59
  Bottom 0.61: v87.22,109.59 87.22,111.97 R66.1
N$52
  Top 0.61: D27.C 87.32,114.62 DRVPWR4.3 87.19,116.93 85.98,116.93 85.09,117.82 D26.C
N$53  (via drill 0.36 pad 0.25, 0.6)
  Top 0.61: DRVPWR4.2 87.78,118.76 87.81,118.79 88.97,118.79 89.51,118.25 89.51,109.95 DRV-I1.2 87.29,107.72 81.98,107.72 81.18,108.53 v28.75,108.53 | v14.09,108.6 11.17,108.6 8.35,111.42 8.35,158.26 13.69,163.59 16.74,163.59 22.88,169.74 DRV_U$7.2
  Bottom 0.61: 87.07,107.51 DRV-I1.2 | v14.09,108.6 28.67,108.6 v28.75,108.53
N$55
  Top 0.305: U6OUT.2 69.57,97.9 U$6.3
  Bottom 0.61: U$6.3 70.91,97.62 R64.2
N$58
  Top 0.305: U$8.8 68.1,88.6 R68.1 66.6,88.63 66.6,89.27 66.75,89.42 67.59,89.42 67.98,89.82 C80.1
R13  (via drill 0.2, 0.5)
  Top 0.254: MSP430F67791A.32 125.26,117.88 126.76,119.38 127.25,119.88 v128,119.88 v128.01,119.88 | R46.2 v132.26,125.38 R43.1
  Bottom 0.254: v132.26,125.38 132.26,123.36 128.88,119.98 128.11,119.98 v128.01,119.88
R23  (via drill 0.2, 0.5)
  Top 0.254: MSP430F67791A.31 125.51,117.38 126.51,118.38 v128.01,118.38 | R43.2 v132.26,121.38 R42.1
  Bottom 0.254: v132.26,121.38 132.26,121.33 129.39,118.46 128.09,118.46 v128.01,118.38
R33  (via drill 0.2, 0.5)
  Top 0.254: MSP430F67791A.30 126.51,116.88 v127.01,117.38 | v132.26,117.38 R42.2 133.16,118.53 133.88,119.25 C49.1
  Bottom 0.254: v127.01,117.38 v132.26,117.38
RESET  (via drill 0.2)
  Top 0.254: C53.2 33.66,141.81 | RESET.1 38.15,140.05 36.91,141.29 33.79,141.29 C53.2 | C53.2 32.32,141.41 31.68,140.76 31.68,140.06 31.67,140.06
  Top 0.305: C53.2 R51.2 | v31.67,135.06 31.67,140.06
  Bottom 0.254: v31.67,135.06 30.67,134.06 26.17,134.06 25.42,134.81 25.42,137.06 24.4,138.08 JP5.3 22.9,138.08 19.18,141.8 | JTAG.11 14.66,140.63 15.83,141.8 19.18,141.8 | 19.18,141.8 19.18,141.81
S0
  Top 0.254: MSP430F67791A.87 101.01,109.88 94.01,116.88 94.01,129.38 91.01,132.38 62.74,132.38 53.58,141.53 LCD1.1
S1
  Top 0.254: MSP430F67791A.86 101.26,110.38 94.51,117.12 94.51,129.62 91.26,132.88 64.76,132.88 56.1,141.53 LCD1.2
S2
  Top 0.254: MSP430F67791A.85 101.51,110.88 95.01,117.38 95.01,129.88 91.51,133.38 66.76,133.38 58.6,141.53 LCD1.3
S3
  Top 0.254: MSP430F67791A.84 101.76,111.38 95.51,117.62 95.51,130.12 91.76,133.88 68.76,133.88 LCD1.4
S4
  Top 0.254: MSP430F67791A.83 102.01,111.88 96.01,117.88 96.01,130.38 92.01,134.38 70.76,134.38 63.64,141.49 LCD1.5
S5
  Top 0.254: MSP430F67791A.82 102.26,112.38 96.51,118.12 96.51,130.62 92.26,134.88 72.76,134.88 66.18,141.45 LCD1.6
S6
  Top 0.254: MSP430F67791A.81 102.51,112.88 97.01,118.38 97.01,130.88 92.51,135.38 74.76,135.38 68.72,141.41 LCD1.7
S7
  Top 0.254: MSP430F67791A.80 102.76,113.38 97.51,118.62 97.51,131.12 92.76,135.88 76.76,135.88 71.26,141.37 LCD1.8
S8
  Top 0.254: MSP430F67791A.79 103.01,113.88 98.01,118.88 98.01,131.38 93.01,136.38 78.76,136.38 73.8,141.33 LCD1.9
S9
  Top 0.254: MSP430F67791A.78 103.26,114.38 98.51,119.12 98.51,131.62 93.26,136.88 80.76,136.88 76.34,141.29 LCD1.10
S10
  Top 0.254: MSP430F67791A.77 103.51,114.88 99.01,119.38 99.01,131.88 93.51,137.38 82.76,137.38 78.88,141.25 LCD1.11
S11
  Top 0.254: MSP430F67791A.76 103.76,115.38 99.51,119.62 99.51,132.12 93.76,137.88 84.76,137.88 81.42,141.21 LCD1.12
S12
  Top 0.254: MSP430F67791A.75 104.01,115.88 100.01,119.88 100.01,132.38 94.01,138.38 86.76,138.38 83.96,141.2 LCD1.13
S13
  Top 0.254: MSP430F67791A.74 104.26,116.38 100.51,120.12 100.51,132.62 94.26,138.88 88.76,138.88 86.5,141.13 LCD1.14
S14
  Top 0.254: MSP430F67791A.73 104.51,116.88 101.01,120.38 101.01,132.88 94.51,139.38 90.76,139.38 89.04,141.12 LCD1.15
S15
  Top 0.254: MSP430F67791A.72 104.76,117.38 101.51,120.62 101.51,133.12 94.76,139.88 92.76,139.88 91.58,141.08 LCD1.16
S16
  Top 0.254: MSP430F67791A.71 105.01,117.88 102.01,120.88 102.01,133.38 94.12,141.29 LCD1.17
S17
  Top 0.254: MSP430F67791A.68 104.26,119.38 102.51,121.12 102.51,133.62 96.66,139.43 LCD1.18
S18
  Top 0.254: MSP430F67791A.67 104.51,119.88 103.01,121.38 103.01,133.88 99.2,137.71 LCD1.19
S19
  Top 0.254: MSP430F67791A.66 104.76,120.38 103.51,121.62 103.51,134.12 101.74,135.92 LCD1.20
S20
  Top 0.254: MSP430F67791A.65 105.01,120.88 104.01,121.88 104.01,141.26 LCD1.21
S21
  Top 0.254: MSP430F67791A.64 109.51,140.88 109.01,141.38 108.81,141.57 106.86,141.57 LCD1.22
S22  (via drill 0.36)
  Top 0.254: MSP430F67791A.63 110.01,141.38 107.01,144.38 v106.51,144.38
  Bottom 0.254: v106.51,144.38 106.51,171.19 LCD1.23
S23  (via drill 0.36)
  Top 0.254: MSP430F67791A.62 110.51,141.62 106.76,145.38 v105.51,145.38
  Bottom 0.254: v105.51,145.38 105.51,170.28 LCD1.24
S24  (via drill 0.36)
  Top 0.254: MSP430F67791A.61 111.01,141.88 106.51,146.38 v104.51,146.38
  Bottom 0.254: v104.51,146.38 104.51,158.38 91.58,171.26 LCD1.29
S25  (via drill 0.36)
  Top 0.254: MSP430F67791A.60 111.51,142.12 106.26,147.38 v103.51,147.38
  Bottom 0.254: v103.51,147.38 103.51,158.62 93.26,168.88 91.51,168.88 89.04,171.34 LCD1.30
S26  (via drill 0.36)
  Top 0.254: MSP430F67791A.59 112.01,142.38 106.01,148.38 v102.51,148.38
  Bottom 0.254: v102.51,148.38 102.51,158.88 93.01,168.38 89.51,168.38 86.5,171.38 LCD1.31
S27  (via drill 0.36)
  Top 0.254: MSP430F67791A.58 112.51,142.62 105.76,149.38 v101.51,149.38
  Bottom 0.254: v101.51,149.38 101.51,159.12 92.76,167.88 87.51,167.88 83.96,171.42 LCD1.32
S28  (via drill 0.36)
  Top 0.254: MSP430F67791A.57 113.01,142.88 105.51,150.38 v100.51,150.38
  Bottom 0.254: v100.51,150.38 100.51,159.38 92.51,167.38 85.51,167.38 81.42,171.46 LCD1.33
S29  (via drill 0.36)
  Top 0.254: MSP430F67791A.56 113.51,143.12 105.26,151.38 v99.51,151.38
  Bottom 0.254: v99.51,151.38 99.51,159.62 92.26,166.88 83.51,166.88 LCD1.34
S30  (via drill 0.36)
  Top 0.254: MSP430F67791A.55 114.01,143.38 105.01,152.38 v98.51,152.38
  Bottom 0.254: v98.51,152.38 98.51,159.88 92.01,166.38 81.51,166.38 76.38,171.5 LCD1.35
S31  (via drill 0.36)
  Top 0.254: MSP430F67791A.54 114.51,143.62 104.76,153.38 v97.51,153.38
  Bottom 0.254: v97.51,153.38 97.51,160.12 91.76,165.88 79.51,165.88 73.88,171.5 LCD1.36
S32  (via drill 0.36)
  Top 0.254: MSP430F67791A.53 115.01,143.88 104.51,154.38 v96.51,154.38
  Bottom 0.254: v96.51,154.38 96.51,160.38 91.51,165.38 77.51,165.38 71.38,171.5 LCD1.37
S33  (via drill 0.36)
  Top 0.254: MSP430F67791A.52 115.51,144.12 104.26,155.38 v95.51,155.38
  Bottom 0.254: v95.51,155.38 95.51,160.62 91.26,164.88 75.51,164.88 68.88,171.5 LCD1.38
S34  (via drill 0.36)
  Top 0.254: MSP430F67791A.51 116.01,144.38 104.01,156.38 v94.51,156.38
  Bottom 0.254: v94.51,156.38 94.51,160.88 91.01,164.38 73.26,164.38 66.18,171.45 LCD1.39
S35  (via drill 0.36)
  Top 0.254: MSP430F67791A.50 116.51,144.62 103.76,157.38 v93.51,157.38
  Bottom 0.254: v93.51,157.38 93.51,161.12 90.76,163.88 71.26,163.88 LCD1.40
S36  (via drill 0.36)
  Top 0.254: MSP430F67791A.49 117.01,144.88 103.51,158.38 v92.51,158.38
  Bottom 0.254: v92.51,158.38 92.51,161.38 90.51,163.38 69.26,163.38 61.13,171.5 LCD1.41
S37  (via drill 0.36)
  Top 0.254: MSP430F67791A.48 117.51,145.12 103.26,159.38 v91.51,159.38
  Bottom 0.254: v91.51,159.38 91.51,161.62 90.26,162.88 67.26,162.88 58.63,171.5 LCD1.42
S38  (via drill 0.36)
  Top 0.254: MSP430F67791A.47 118.01,145.38 103.01,160.38 v90.51,160.38
  Bottom 0.254: v90.51,160.38 90.51,161.88 90.01,162.38 65.26,162.38 56.13,171.5 LCD1.43
S39  (via drill 0.36)
  Top 0.254: MSP430F67791A.46 118.51,145.62 102.76,161.38 v89.51,161.38
  Bottom 0.254: v89.51,161.38 89.01,161.88 63.01,161.88 53.48,171.4 LCD1.44
TCK
  Top 0.254: R48.1 21.62,140.09 22.14,140.62 JP6.3
  Bottom 0.254: JP6.3 22.91,140.62 19.1,144.43 15.92,144.43 JTAG.7
TDI
  Bottom 0.254: JP8.3 22.91,145.7 19.05,149.56 15.88,149.56 JTAG.3
TDO
  Top 0.254: JP9.3 25.45,146.97 27.36,146.97 27.99,146.33 27.99,139.35 JP5.1
  Bottom 0.254: JP9.3 22.91,148.24 19.1,152.05 15.93,152.05 JTAG.1
TEST/SBWTCK  (via drill 0.36)
  Top 0.254: JTAG.8 19.1,143.79 19.1,135.54 20.37,134.27 22.91,134.27 JP4.3 JP4.2 26.72,135.51 27.82,134.41 28.17,134.06 28.2,134.03 33.27,134.03 36.12,136.88 55.54,136.88 60.58,131.83 90.76,131.88 93.51,129.12 93.51,116.12 94.55,115.08 v94.74,115.08 | MSP430F67791A.97 101.51,104.88 v100.88,104.25
  Bottom 0.254: v100.88,104.25 100.81,104.18 99.06,104.18 95.25,107.99 95.25,114.57 v94.74,115.08
TMS
  Bottom 0.254: JP7.3 22.91,143.16 19.14,146.93 15.96,146.93 JTAG.5
VASYS1/2
  Top 0.254: C23.1 112.01,94.12 111.86,93.97 C22.1 110.51,94.88 113.51,97.88 MSP430F67791A.111 113.51,101.47 112.8,102.18 112.8,102.53 113.14,102.88 118.51,102.88 119.01,102.38 MSP430F67791A.122 119.01,98.48 120.61,96.88 122.51,96.88 122.75,96.64 C32.1
  Top 0.406: C32.1 122.75,95.64 122.76,95.62 C28.1
VCORE
  Top 0.254: C38.1 123.51,100.38 123.51,100.58 MSP430F67791A.128
VREF
  Top 0.254: C30.1 115.11,98.83 114.51,99.43 MSP430F67791A.113
XIN
  Top 0.254: MSP430F67791A.1 126.01,102.38 126.86,101.53 128.41,101.53 XT1.P2 130.51,101.38 131.41,100.47 C37.1 131.41,99.97
XOUT
  Top 0.254: XT1.P1 128.41,104.06 | MSP430F67791A.2 126.01,102.88 127.01,103.88 XT1.P1 | XT1.P1 130.55,103.88 131.37,104.69 131.37,105.34 C40.1

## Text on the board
tNames: + | + | + | + | + | + | + | + | M. MESGANAW / MARCH 2017 | DVCC | INTERNAL | EXTERNAL | TIDA-01377 | J=JTAG | J | S | S=SBW | Version 1.1, 2 coil set implementation | GND | VDD | ENABLE | OUT | AUXVCC1 | AUXVCC2 | AUXVCC3 | DGND | DGND | VDSYS | REF | SENSE | COM | GND
_tplace: C1 | U$7 | DVCC | DRV_U$7 | R1 | DGND | 1 | LED3 | LED2 | LED1 | LED_A | LED_B | LED4 | LED5 | LED6 | R54 | + | R55 | + | R56 | + | R57 | + | R58 | + | R59 | + | R60 | + | R61 | + | M. MESGANAW / MARCH 2017 | DVCC | 1 | 2 | INTERNAL | EXTERNAL | RESET | TIDA-01377 | 14 | LCD1 | R51 | DBTN2 | DBTN1 | R48 | C53 | J=JTAG | J | S | S=SBW | R53 | JTAG | R50 | LDIG | Version 1.1, 2 coil set implementation | R46 | LDC_PWR | GND | LED7 | C58 | VDD | R4 | C36 | D26 | R43 | ENABLE | C49 | OUT | R42 | 1 | DRVPWR4 | D27 | MSP430F67791A | C43 | C44 | C40 | DRV-I1 | 1 | U$6 | C38 | XT1 | C34 | C35 | C37 | U6GND | C30 | C33 | U4GND | 1 | U6OUT | C31 | C32 | 1 | C22 | C23 | C29 | C28 | C52 | C15 | R15 | 1 | C24 | C25 | C26 | C27 | AUXVCC1 | AUXVCC2 | AUXVCC3 | U5OUT | R45 | 1 | C80 | C14 | 1 | D44 | 1 | U$5 | R68 | U$4 | U$8 | 1 | R36 | DGND | DGND | VDSYS | 1 | 1 | R16 | U5GND | U4OUT | HD1 | C12 | R17 | AD_SEL | 1 | EN_SEL | 1 | R10 | R9 | U1 | R13 | REF | SENSE | R12 | C9 | C10 | C11 | R11 | COM | LANLG | GND
_bplace: R8 | R66 | C55 | R64 | R47 | C54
